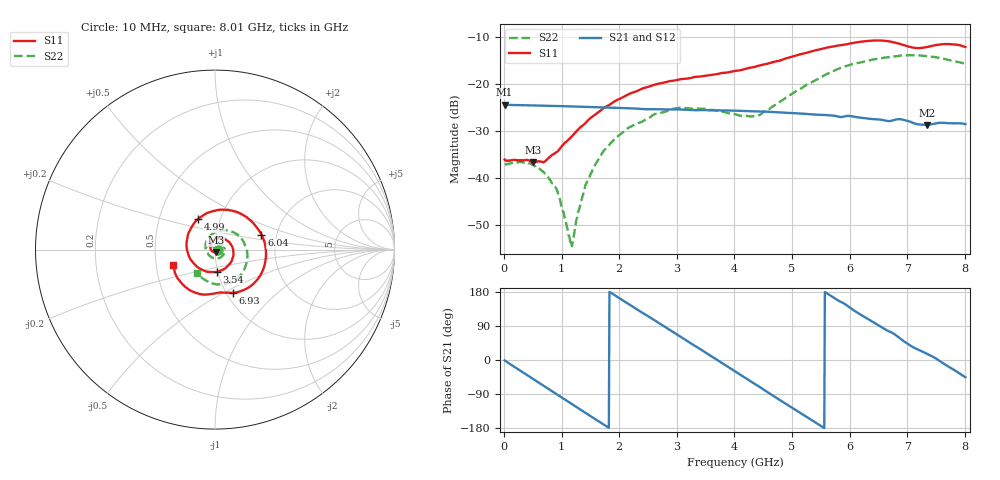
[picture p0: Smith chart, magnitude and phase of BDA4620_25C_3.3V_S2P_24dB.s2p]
!Agilent Technologies,E5071B,MY42404982,A.09.10
!Date: Wed May 06 08:54:01 2026
!Data & Calibration Information:
!Freq	S11:SOLT2(ON)	S21:SOLT2(ON)	S12:SOLT2(ON)	S22:SOLT2(ON)
# Hz S RI R 50
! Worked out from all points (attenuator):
!   801 points, 10 MHz to 8.01 GHz, reference 50 ohm
!   highest |S21| = -24.39 dB at 10 MHz (marker M1); lowest = -28.7 dB at 7.34 GHz (marker M2)
!   lowest |S11| = -36.7 dB at 510 MHz (marker M3), VSWR 1.03, Z = 50.3 - j1.43 ohm
!   |S11| at or under -10 dB: start of sweep to end of sweep
!   |S22| runs from -54.4 to -13.9 dB; largest |S21 - S12| = 0.00028
!   S11 on the Smith chart (normalised r, x): 10 MHz: 1.03, -0.00; 3.54 GHz: 0.99, -0.25; 4.99 GHz: 0.78, +0.28; 6.04 GHz: 1.67, +0.30; 6.93 GHz: 1.08, -0.55; 8.01 GHz: 0.62, -0.11
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1e7  0.0158 -0.00109  0.0603 -0.00126  0.0604 -0.00126  0.014 -0.000438
5.1e8  0.00362 -0.0142  0.0374 -0.046  0.0375 -0.0461  0.0125 -0.00564
8.9e8  -0.0165 -0.00856  0.0017 -0.0585  0.00168 -0.0586  0.00419 -0.00687
1.16e9  -0.0254 0.00936  -0.0243 -0.0525  -0.0244 -0.0526  -0.0016 -0.00113
1.2e9  -0.026 0.0126  -0.0278 -0.0507  -0.0279 -0.0508  -0.0022 -3.46e-05
1.35e9  -0.0252 0.0253  -0.0395 -0.0417  -0.0395 -0.0418  -0.00375 0.00466
1.53e9  -0.018 0.0411  -0.0498 -0.0277  -0.0498 -0.0278  -0.00356 0.0114
1.77e9  0.00173 0.0574  -0.056 -0.0057  -0.0562 -0.00572  0.000635 0.0207
2.14e9  0.0473 0.0604  -0.0479 0.0279  -0.048 0.0279  0.0167 0.0292
2.68e9  0.1007 0.00286  -0.00789 0.0535  -0.00788 0.0535  0.0446 0.0195
3.54e9  0.012 -0.123  0.0508 0.0142  0.0508 0.0141  0.0356 -0.0402
4.01e9  -0.0972 -0.0976  0.0452 -0.026  0.0453 -0.026  -0.0106 -0.0468
4.42e9  -0.1565 0.00185  0.0179 -0.0479  0.0179 -0.0479  -0.0448 -0.0129
4.99e9  -0.0949 0.1695  -0.0283 -0.0404  -0.0283 -0.0404  -0.0326 0.0711
5.35e9  0.0274 0.222  -0.0447 -0.0165  -0.0447 -0.0166  0.0229 0.1024
6.04e9  0.2591 0.0829  -0.0317 0.0325  -0.0318 0.0326  0.1528 0.0545
6.36e9  0.2807 -0.065  -0.0106 0.0413  -0.0106 0.0413  0.1788 -0.0134
6.68e9  0.2015 -0.2012  0.00986 0.0393  0.00987 0.0393  0.1707 -0.0906
6.93e9  0.1005 -0.2405  0.0264 0.0323  0.0265 0.0324  0.1396 -0.1457
7.34e9  -0.0146 -0.2466  0.0353 0.0106  0.0354 0.0106  0.0426 -0.1938
7.66e9  -0.1426 -0.2251  0.0377 -0.00817  0.0378 -0.00818  -0.0359 -0.181
8.01e9  -0.2315 -0.0876  0.0263 -0.0267  0.0264 -0.0268  -0.1026 -0.1278
